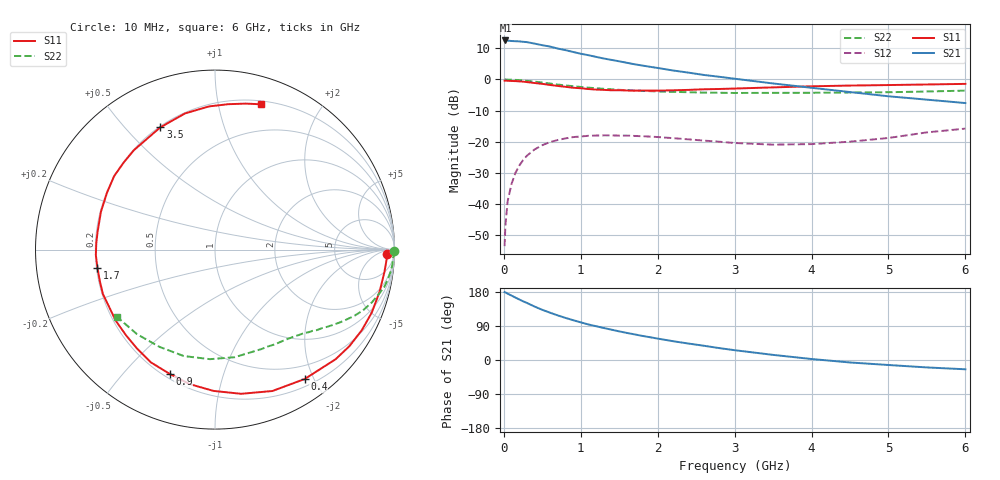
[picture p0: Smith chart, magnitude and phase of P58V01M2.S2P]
! SIEMENS Small Signal Semiconductors
! BFP183
! Si NPN RF Bipolar Junction Transistor in SOT143
! VCE = 8 V  IC = 1.2 mA
! Common Emitter S-Parameters:  March  1996
# GHz  S  MA  R  50
!  f  S11  S21  S12  S22
! GHz  MAG  ANG  MAG  ANG  MAG  ANG  MAG  ANG
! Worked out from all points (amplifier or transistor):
!   36 points, 10 MHz to 6 GHz, reference 50 ohm
!   highest |S21| = 12.5 dB at 20 MHz (marker M1)
!   |S21| within 3 dB of that: start of sweep to 780.5 MHz
!   unconditionally stable (mu >= 1): 2.461 GHz to end of sweep
!   at 250 MHz: K = 0.10, MSG = 19.0 dB, |S12| = -25.9 dB
!   at 1.4 GHz: K = 0.55, MSG = 12.1 dB, |S12| = -18.0 dB
!   at 6 GHz: K = 1.02, MAG = 3.3 dB, |S12| = -15.8 dB
!   S11 on the Smith chart (normalised r, x): 10 MHz: 35, -20; 400 MHz: 0.30, -1.87; 900 MHz: 0.22, -0.68; 1.7 GHz: 0.20, -0.07; 3.5 GHz: 0.20, +0.63; 6 GHz: 0.23, +1.34
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0.01  0.9579 -1.4  4.213 179.2  0.0021 84.5  1 -0.5
0.02  0.9586 -2.9  4.234 178.5  0.0045 86.1  0.9999 -1.1
0.05  0.9521 -7.5  4.207 175.0  0.0112 87.0  0.9936 -2.5
0.1  0.9467 -14.3  4.149 170.0  0.021 80.7  0.9913 -5.1
0.15  0.9413 -21.9  4.118 164.8  0.0314 77.0  0.9845 -7.6
0.25  0.9222 -35.6  4.032 154.9  0.0506 69.0  0.9659 -12.4
0.3  0.9081 -42.3  3.982 150.6  0.0596 64.9  0.9505 -14.5
0.4  0.8771 -55.3  3.767 141.0  0.0753 57.7  0.923 -18.5
0.5  0.8503 -67.9  3.55 132.4  0.088 50.5  0.8917 -22.3
0.6  0.8166 -79.7  3.377 124.9  0.0987 44.4  0.8597 -25.4
0.7  0.7874 -90.6  3.14 117.7  0.1065 39.0  0.8289 -28.1
0.8  0.7626 -100.7  2.964 111.2  0.1131 34.0  0.8025 -30.5
0.9  0.7368 -110.1  2.766 105.1  0.1186 29.6  0.7791 -32.6
1.1  0.7016 -128.4  2.454 93.8  0.1245 21.9  0.7383 -36.4
1.4  0.6709 -151.4  2.062 80.0  0.1264 13.1  0.6953 -41.5
1.7  0.6625 -171.3  1.753 67.6  0.1238 6.7  0.6637 -46.1
2.2  0.6696 161.7  1.394 49.6  0.1141 0.3  0.6321 -54.0
2.8  0.7032 136.2  1.105 31.4  0.1 -1.0  0.6117 -64.9
3.5  0.7462 114.1  0.863 13.5  0.0898 6.0  0.6095 -79.7
4.5  0.7985 92.4  0.628 -6.5  0.1002 21.2  0.6181 -106.3
5.5  0.8309 78.2  0.474 -19.6  0.1413 26.8  0.6409 -132.7
6  0.8495 72.4  0.418 -24.5  0.1624 23.9  0.6618 -145.4
